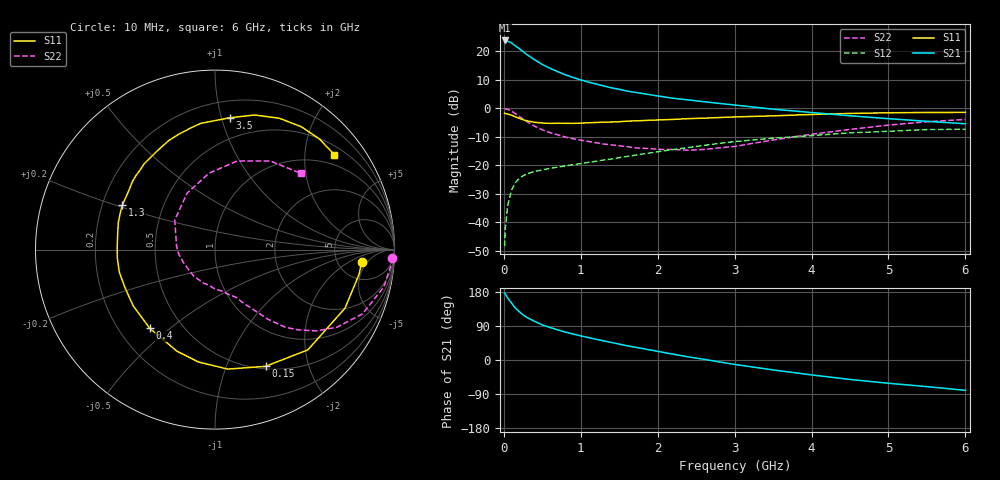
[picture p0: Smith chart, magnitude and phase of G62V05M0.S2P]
! SIEMENS Small Signal Semiconductors
! BFG193
! Si NPN RF Bipolar Junction Transistor in SOT223
! VCE = 2 V  IC = 5 mA
! Common Emitter S-Parameters:  August  1996
# GHz  S  MA  R  50
!  f  S11  S21  S12  S22
! GHz  MAG  ANG  MAG  ANG  MAG  ANG  MAG  ANG
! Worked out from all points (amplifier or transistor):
!   36 points, 10 MHz to 6 GHz, reference 50 ohm
!   highest |S21| = 23.9 dB at 10 MHz (marker M1)
!   |S21| within 3 dB of that: start of sweep to 206.6 MHz
!   unconditionally stable (mu >= 1): 1.105 GHz to 2.683 GHz
!   at 250 MHz: K = 0.34, MSG = 21.8 dB, |S12| = -23.7 dB
!   at 1.4 GHz: K = 1.09, MAG = 10.6 dB, |S12| = -17.8 dB
!   at 6 GHz: K = 0.92, MSG = 1.0 dB, |S12| = -7.4 dB
!   S11 on the Smith chart (normalised r, x): 10 MHz: 8.46, -3.68; 150 MHz: 0.53, -1.38; 400 MHz: 0.33, -0.43; 1.3 GHz: 0.28, +0.21; 3.5 GHz: 0.33, +1.06; 6 GHz: 0.71, +2.70
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0.01  0.8196 -5.0  15.59 176.5  0.0038 92.8  0.9884 -2.6
0.02  0.8144 -9.8  15.53 174.2  0.0081 84.3  0.9848 -5.1
0.05  0.7943 -24.3  15.16 163.4  0.0198 77.5  0.9632 -12.5
0.1  0.7613 -47.2  14.1 150.2  0.0366 67.7  0.8966 -23.5
0.15  0.7087 -66.6  12.5 136.9  0.0495 57.6  0.8051 -32.5
0.2  0.6696 -83.9  11.22 127.6  0.0592 52.2  0.7245 -38.7
0.25  0.6331 -98.3  9.928 118.9  0.0655 47.0  0.6436 -44.0
0.3  0.6046 -110.5  8.808 112.3  0.0708 43.8  0.5843 -47.8
0.4  0.5696 -129.6  7.137 101.9  0.0781 39.2  0.4869 -52.8
0.5  0.5531 -145.5  5.906 92.7  0.083 36.9  0.4202 -56.0
0.6  0.5445 -156.9  5.07 85.8  0.0884 36.0  0.376 -58.8
0.7  0.5479 -166.7  4.419 79.4  0.0927 35.9  0.3432 -61.6
0.9  0.5451 177.6  3.489 68.5  0.1028 35.8  0.2928 -65.9
1.1  0.559 164.6  2.895 59.1  0.1126 36.1  0.2623 -72.9
1.3  0.5731 154.3  2.476 50.4  0.1241 36.2  0.2363 -79.4
1.6  0.596 140.6  2.02 37.6  0.1431 34.9  0.2129 -93.3
2.2  0.64 119.3  1.507 15.4  0.1892 29.3  0.1898 -128.3
2.8  0.69 101.6  1.223 -5.0  0.2431 19.8  0.2024 -171.6
3.5  0.7388 83.7  0.968 -26.2  0.2996 4.7  0.2783 143.7
4.5  0.8149 63.9  0.741 -51.3  0.3721 -15.5  0.4275 94.4
5.5  0.8477 46.7  0.593 -70.3  0.4247 -40.5  0.5823 58.0
6  0.8496 38.5  0.536 -80.0  0.429 -54.6  0.6393 41.7
